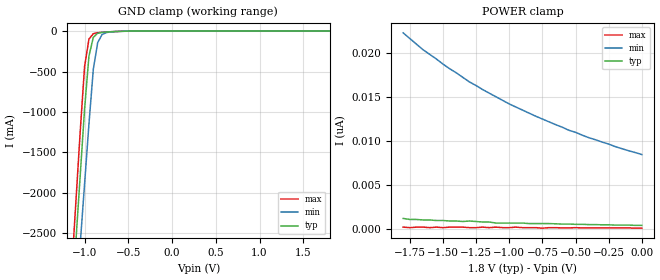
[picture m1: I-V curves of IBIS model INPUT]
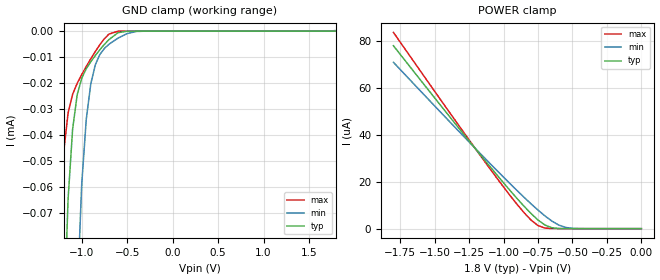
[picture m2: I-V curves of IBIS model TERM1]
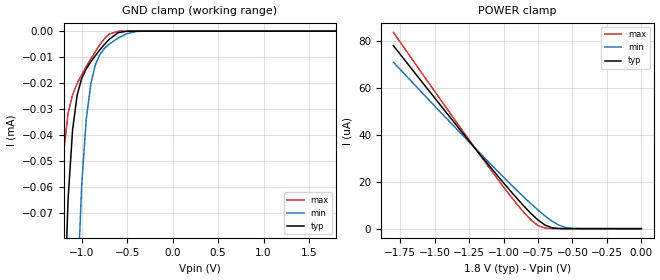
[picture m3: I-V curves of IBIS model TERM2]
|   DIODES INCORPORATED
|   IBIS Model of PI2SSD3212
|   Product Family: 2SSD
|   TQFN (ZL) Package
[IBIS Ver] 4.0
[Comment char] |_char
[File Name] pi2ssd3212_zl_18v.ibs
[File Rev] 1.0
[Source] File originated at Diodes Incorporated.
[Date] 04/22/19
[Disclaimer] (C) Copyright DIODES INCORPORATED
   All rights reserved
  Diodes Incorporated hereby grants the user of
  this IBIS model a non-exclusive, nontransferable license to
  use this IBIS model under the following terms.
  This IBIS model is provided on an "AS IS" basis and Diodes
  makes absolutely no warranty with respect to the information
  contained herein. DIODES DISCLAIMS AND CUSTOMER WAIVES ALL
  WARRANTIES, EXPRESSED OR IMPLIED, INCLUDING WARRANTIES OF
  MERCHANTABILITY OR FITNESS FOR A PARTICULAR PURPOSE. The
  entire risk as to quality and performance is with the customer.
  Accordingly, in no event shall the company be liable for any
  damages, whether in contract or tort, including any lost
  profits or other incidental, consequential, exemplary, or
  punitive damages arising out of the use or application of the
  IBIS model provided in this package. Further, Diodes reserves
  the right to make changes without notice to any product herein
  to improve reliability, function, or design. Diodes does not
  convey any license under patent rights or any other intellectual
  property rights, including those of third parties.
  The user is granted this license only to use the IBIS model
  and is not granted rights to sell, load, rent, lease or license
  the IBIS model in whole or in part, or in modified form to anyone
  other than user. User may modify the IBIS model to suit its specific
  application but rights to derivative works and such modifications
  shall belong to Diodes.
  Diodes is not obligated to provide maintenance or support
  for the licensed IBIS model.
  Contact Diodes at ATTN: APPLICATION ENGINEERING / IBIS MODELS
  1545 Barber Lane Milpitas, CA 95035 USA.
[Component] PI2SSD3212
[Manufacturer] Diodes Incorporated.
[Package]
| variable   typ   min   max
R_pkg   0.03902ohm   0.02922ohm   0.06842ohm
L_pkg   0.79998nH   0.76828nH   0.89508nH
C_pkg   0.19606pF   0.17176pF   0.26896pF
[Pin]   signal_name   model_name   R_pin   L_pin   C_pin
1   GND   GND   0.06842   0.89508nH   0.26896pF
2   EN   INPUT   0.06450   0.88240nH   0.25924pF
3   A13   TERM1   0.06058   0.86972nH   0.24952pF
4   A12   TERM1   0.05666   0.85704nH   0.23980pF
5   A11   TERM1   0.05274   0.84436nH   0.23008pF
6   VDD   POWER   0.04882   0.83168nH   0.22036pF
7   A10   TERM1   0.04490   0.81900nH   0.21064pF
8   A9   TERM1   0.04098   0.80632nH   0.20092pF
9   A8   TERM1   0.03706   0.79364nH   0.19120pF
10   A7   TERM1   0.03314   0.78096nH   0.18148pF
11   GND   GND   0.02922   0.76828nH   0.17176pF
12   A6   TERM1   0.03314   0.78096nH   0.18148pF
13   A5   TERM1   0.03706   0.79364nH   0.19120pF
14   A4   TERM1   0.04098   0.80632nH   0.20092pF
15   A3   TERM1   0.04490   0.81900nH   0.21064pF
16   GND   GND   0.04882   0.83168nH   0.22036pF
17   A2   TERM1   0.05274   0.84436nH   0.23008pF
18   A1   TERM1   0.05666   0.85704nH   0.23980pF
19   A0   TERM1   0.06058   0.86972nH   0.24952pF
20   SEL   INPUT   0.06450   0.88240nH   0.25924pF
21   GND   GND   0.06842   0.89508nH   0.26896pF
22   C0   TERM2   0.03706   0.79364nH   0.19120pF
23   B0   TERM2   0.03314   0.78096nH   0.18148pF
24   C1   TERM2   0.02922   0.76828nH   0.17176pF
25   B1   TERM2   0.03314   0.78096nH   0.18148pF
26   GND   GND   0.03706   0.79364nH   0.19120pF
27   C2   TERM2   0.06842   0.89508nH   0.26896pF
28   B2   TERM2   0.06450   0.88240nH   0.25924pF
29   C3   TERM2   0.06058   0.86972nH   0.24952pF
30   B3   TERM2   0.05666   0.85704nH   0.23980pF
31   C4   TERM2   0.05274   0.84436nH   0.23008pF
32   B4   TERM2   0.04882   0.83168nH   0.22036pF
33   C5   TERM2   0.04490   0.81900nH   0.21064pF
34   B5   TERM2   0.04098   0.80632nH   0.20092pF
35   C6   TERM2   0.03706   0.79364nH   0.19120pF
36   B6   TERM2   0.03314   0.78096nH   0.18148pF
37   VDD   POWER   0.02922   0.76828nH   0.17176pF
38   C7   TERM2   0.03314   0.78096nH   0.18148pF
39   B7   TERM2   0.03706   0.79364nH   0.19120pF
40   C8   TERM2   0.04098   0.80632nH   0.20092pF
41   B8   TERM2   0.04490   0.81900nH   0.21064pF
42   C9   TERM2   0.04882   0.83168nH   0.22036pF
43   B9   TERM2   0.05274   0.84436nH   0.23008pF
44   C10   TERM2   0.05666   0.85704nH   0.23980pF
45   B10   TERM2   0.06058   0.86972nH   0.24952pF
46   C11   TERM2   0.06450   0.88240nH   0.25924pF
47   B11   TERM2   0.06842   0.89508nH   0.26896pF
48   GND   GND   0.03706   0.79364nH   0.19120pF
49   C12   TERM2   0.03314   0.78096nH   0.18148pF
50   B12   TERM2   0.02922   0.76828nH   0.17176pF
51   C13   TERM2   0.03314   0.78096nH   0.18148pF
52   B13   TERM2   0.03706   0.79364nH   0.19120pF
[Series Switch Groups]
On 1 /
Off 2 /
[Series Pin Mapping]   pin_2   model_name  function_table_group
19   23   SWITCH1   1
18   25   SWITCH1   1
17   28   SWITCH1   1
15   30   SWITCH1   1
14   32   SWITCH1   1
13   34   SWITCH1   1
12   36   SWITCH1   1
10   39   SWITCH1   1
9   41   SWITCH1   1
8   43   SWITCH1   1
7   45   SWITCH1   1
5   47   SWITCH1   1
4   50   SWITCH1   1
3   52   SWITCH1   1
19   22   SWITCH1   2
18   24   SWITCH1   2
17   27   SWITCH1   2
15   29   SWITCH1   2
14   31   SWITCH1   2
13   33   SWITCH1   2
12   35   SWITCH1   2
10   38   SWITCH1   2
9   40   SWITCH1   2
8   42   SWITCH1   2
7   44   SWITCH1   2
5   46   SWITCH1   2
4   49   SWITCH1   2
3   51   SWITCH1   2
|   Model SWITCH1
[Model] SWITCH1
Model_type Series_switch
| variable   typ   min   max
C_comp   1.1408pF   0.7359pF   1.2215pF
[Voltage Range]   1.8000V   1.6200V   1.9800V
[GND Clamp Reference]   0.0000V   0.0000V   0.0000V
[POWER Clamp Reference]   1.8000V   1.6200V   1.9800V
[Temperature Range]   25   85   -10
[On]
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[OFF]
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| Models and submodels in the file (4): INPUT (Input), SWITCH1 (Series_switch), TERM1 (Terminator), TERM2 (Terminator)
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|   Model INPUT
[Model] INPUT
Model_type Input
Vinl = 800mV
Vinh = 2.0V
| variable   typ   min   max
C_comp   1.6846pF   1.6844pF   1.6848pF
[Voltage Range]   1.8000V   1.6200V   1.9800V
[GND Clamp Reference]   0.0000V   0.0000V   0.0000V
[POWER Clamp Reference]   1.8000V   1.6200V   1.9800V
[Temperature Range]   25   85   -10
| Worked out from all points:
|   GND clamp passes 1 mA (typ) near -0.51 V on its own axis
[GND Clamp]
| Voltage   I(typ)   I(min)   I(max)
-1.8V     -14.14A    -13.78A    -14.43A
-1.15V    -3.434A    -4.119A    -3.003A
-1.1V     -2.61A     -3.376A    -2.124A
-1.05V    -1.787A    -2.634A    -1.245A
-1V       -963.7mA   -1.891A    -439.9mA
-950mV    -309.6mA   -1.148A    -98.81mA
-900mV    -76.73mA   -470.7mA   -31.85mA
-850mV    -27.09mA   -141.9mA   -19.69mA
-800mV    -16.15mA   -42.85mA   -14.83mA
-750mV    -11.66mA   -17.83mA   -11.13mA
-400mV    -76.03uA   -213.9uA   -33.15uA
1.8V      378.3pA    9.284nA    87.31pA
[POWER Clamp]   |Note: Vtable = Vcc - Voutput
| Voltage   I(typ)   I(min)   I(max)
-1.8V     1.164nA    22.29nA    174.6pA
-1.75V    1.048nA    21.65nA    116.4pA
-1.65V    989.5pA    20.37nA    174.6pA
-1.45V    873.1pA    18.22nA    174.6pA
-1.3V     873.1pA    16.71nA    116.4pA
-1.15V    756.7pA    15.43nA    116.4pA
-1.1V     640.3pA    15.02nA    174.6pA
-1V       640.3pA    14.2nA     116.4pA
-800mV    582.1pA    12.81nA    116.4pA
-550mV    523.9pA    11.21nA    87.31pA
-200mV    407.5pA    9.342nA    87.31pA
0V        378.3pA    8.44nA     58.21pA
|   Model TERM1
[Model] TERM1
Model_type Terminator
| variable   typ   min   max
C_comp   1.2292pF   1.1332pF   1.7052pF
[Voltage Range]   1.8000V   1.6200V   1.9800V
[GND Clamp Reference]   0.0000V   0.0000V   0.0000V
[POWER Clamp Reference]   1.8000V   1.6200V   1.9800V
[Temperature Range]   25   85   -10
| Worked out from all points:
|   GND clamp passes 1 mA (typ) near -1.43 V on its own axis
[GND Clamp]
| Voltage   I(typ)   I(min)   I(max)
-1.8V     -19.99mA   -143.3mA   -6.049mA
-1.25V    -206.7uA   -655.5uA   -81.59uA
-1.2V     -116.4uA   -445uA     -47.23uA
-1.15V    -64.78uA   -286.8uA   -31.56uA
-1.1V     -37.79uA   -175.6uA   -24.36uA
-1.05V    -24.6uA    -103.1uA   -20.14uA
-950mV    -14.48uA   -34.03uA   -13.64uA
-900mV    -11.77uA   -20.3uA    -10.66uA
-800mV    -7.162uA   -8.979uA   -5.205uA
-700mV    -3.234uA   -5.048uA   -1.137uA
-400mV    -516.6pA   -116.9nA   -36.38pA
1.8V      87.31pA    227.1nA    87.31pA
[POWER Clamp]   |Note: Vtable = Vcc - Voutput
| Voltage   I(typ)   I(min)   I(max)
-1.8V     78.1uA     71.01uA    83.78uA
-1.4V     48.38uA    46.17uA    50.24uA
-1.1V     26.57uA    27.89uA    25.66uA
-900mV    12.71uA    16.13uA    10.2uA
-800mV    6.402uA    10.55uA    3.616uA
-750mV    3.672uA    7.912uA    1.307uA
-700mV    1.551uA    5.445uA    250.4nA
-650mV    401.2nA    3.258uA    31.37nA
-600mV    68.83nA    1.541uA    3.696nA
-550mV    10.33nA    515.7nA    465.7pA
-450mV    261.9pA    26.54nA    87.31pA
0V        87.31pA    29.1pA     58.21pA
|   Model TERM2
[Model] TERM2
Model_type Terminator
| variable   typ   min   max
C_comp   1.1332pF   0.5443pF   1.2217pF
[Voltage Range]   1.8000V   1.6200V   1.9800V
[GND Clamp Reference]   0.0000V   0.0000V   0.0000V
[POWER Clamp Reference]   1.8000V   1.6200V   1.9800V
[Temperature Range]   25   85   -10
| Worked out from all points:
|   GND clamp passes 1 mA (typ) near -1.43 V on its own axis
[GND Clamp]
| Voltage   I(typ)   I(min)   I(max)
-1.8V     -15.22mA   -92.46mA   -5.486mA
-1.25V    -205uA     -643.2uA   -81.34uA
-1.2V     -115.8uA   -438.2uA   -47.16uA
-1.15V    -64.59uA   -283.4uA   -31.54uA
-1.1V     -37.73uA   -174.1uA   -24.35uA
-1.05V    -24.58uA   -102.5uA   -20.13uA
-950mV    -14.48uA   -33.95uA   -13.63uA
-900mV    -11.77uA   -20.28uA   -10.65uA
-800mV    -7.16uA    -8.974uA   -5.204uA
-700mV    -3.233uA   -5.046uA   -1.137uA
-400mV    -523.9pA   -116.8nA   -14.55pA
1.8V      0A         227.1nA    0A
[POWER Clamp]   |Note: Vtable = Vcc - Voutput
| Voltage   I(typ)   I(min)   I(max)
-1.8V     78.1uA     71.01uA    83.78uA
-1.4V     48.38uA    46.17uA    50.24uA
-1.1V     26.57uA    27.89uA    25.66uA
-900mV    12.71uA    16.13uA    10.2uA
-800mV    6.402uA    10.55uA    3.616uA
-750mV    3.672uA    7.912uA    1.307uA
-700mV    1.551uA    5.445uA    250.4nA
-650mV    401.2nA    3.258uA    31.37nA
-600mV    68.83nA    1.541uA    3.696nA
-550mV    10.33nA    515.7nA    465.7pA
-450mV    261.9pA    26.54nA    87.31pA
0V        87.31pA    29.1pA     58.21pA
